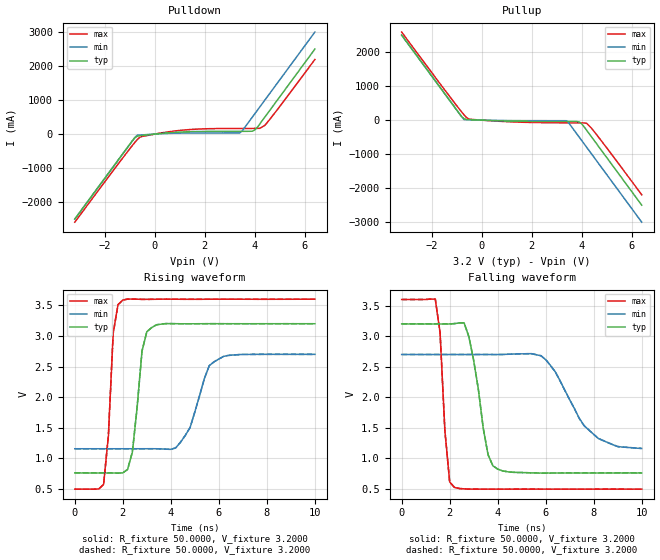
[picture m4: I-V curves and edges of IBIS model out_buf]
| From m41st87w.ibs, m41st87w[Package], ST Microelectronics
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|   Model out_buf
[Model]   out_buf
Model_type   Output
Polarity   Non-Inverting
Vmeas =   1.5000V
Cref =  50.0000pF
Rref =   0.6450k
Vref =   1.7500V
C_comp   9.2400pF   8.7300pF   9.7600pF
[Temperature Range]   27.0000   85.0000   -40.0000
[Voltage Range]   3.2000V   2.7000V   3.6000V
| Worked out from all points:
|   slope of the pulldown table from 0 to 0.48 V, typ, clamps not added: 14.3 ohm
|   slope of the pullup table from 0 to 0.48 V, typ, clamps not added: 36.1 ohm
|   rising waveform, R_fixture 50.0000, V_fixture 3.2000: 20-80 % time 352ps typ, 738ps min, 255ps max; typ from 0.763 V to 3.2 V
|   rising waveform, R_fixture 50.0000, V_fixture 3.2000: 20-80 % time 352ps typ, 738ps min, 255ps max; typ from 0.763 V to 3.2 V
|   falling waveform, R_fixture 50.0000, V_fixture 3.2000: 20-80 % time 568ps typ, 1.35ns min, 271ps max; typ from 3.2 V to 0.763 V
|   falling waveform, R_fixture 50.0000, V_fixture 3.2000: 20-80 % time 568ps typ, 1.35ns min, 271ps max; typ from 3.2 V to 0.763 V
[Pulldown]
| voltage   I(typ)   I(min)   I(max)
-3.2V     -2.5A      -2.5A      -2.591A
-900mV    -200mA     -200mA     -337.2mA
-700mV    -62.82mA   -32.69mA   -160.6mA
-500mV    -39.9mA    -23.29mA   -67.68mA
900mV     54.82mA    27.57mA    99.9mA
3.4V      81.17mA    34.99mA    165.9mA
3.5V      81.34mA    100mA      166.2mA
3.9V      85.33mA    500mA      167.5mA
4V        121.5mA    600mA      167.8mA
4.2V      300mA      800mA      168.7mA
4.4V      500mA      1A         256.9mA
6.4V      2.5A       3A         2.194A
[Pullup]
| voltage   I(typ)   I(min)   I(max)
-3.2V     2.5A       2.5A       2.589A
-900mV    200mA      200mA      332.4mA
-700mV    40.85mA    13.49mA    150.9mA
-500mV    16.27mA    9.076mA    29.84mA
-300mV    9.6mA      5.337mA    16.43mA
1.4V      -30.11mA   -14.05mA   -55.76mA
3.4V      -38.98mA   -17.38mA   -78.6mA
3.9V      -52.76mA   -500mA     -80.59mA
4V        -109mA     -600mA     -80.96mA
4.2V      -300mA     -800mA     -95.49mA
4.6V      -700mA     -1.2A      -430.6mA
6.4V      -2.5A      -3A        -2.194A
[Ramp]
| variable   typ   min   max
dV/dt_r   1.8251/0.5037n   1.4741/1.0410n   2.0984/0.2774n
dV/dt_f   1.8833/0.3740n   1.5639/0.8009n   2.1365/0.1990n
R_load = 0.6450k
[Rising Waveform]
R_fixture = 50.0000
V_fixture = 3.2000
V_fixture_min = 2.7000
V_fixture_max = 3.6000
| time   V(typ)   V(min)   V(max)
0s        762.9mV    1.158V     498.2mV
1.2ns     762.9mV    1.158V     576.1mV
1.6ns     762.9mV    1.158V     3.047V
2ns       763.6mV    1.158V     3.587V
2.4ns     1.105V     1.158V     3.603V
2.8ns     2.755V     1.158V     3.598V
3.2ns     3.136V     1.159V     3.599V
4.4ns     3.199V     1.263V     3.6V
5.8ns     3.201V     2.579V     3.6V
10ns      3.2V       2.7V       3.6V
[Rising Waveform]
R_fixture = 50.0000
V_fixture = 3.2000
V_fixture_min = 2.7000
V_fixture_max = 3.6000
| time   V(typ)   V(min)   V(max)
0s        762.9mV    1.158V     498.2mV
1.2ns     762.9mV    1.158V     576.1mV
1.6ns     762.9mV    1.158V     3.047V
2ns       763.6mV    1.158V     3.587V
2.4ns     1.105V     1.158V     3.603V
2.8ns     2.755V     1.158V     3.598V
3.2ns     3.136V     1.159V     3.599V
4.4ns     3.199V     1.263V     3.6V
5.8ns     3.201V     2.579V     3.6V
10ns      3.2V       2.7V       3.6V
[Falling Waveform]
R_fixture = 50.0000
V_fixture = 3.2000
V_fixture_min = 2.7000
V_fixture_max = 3.6000
| time   V(typ)   V(min)   V(max)
0s        3.2V       2.7V       3.6V
1.4ns     3.2V       2.7V       3.606V
1.6ns     3.2V       2.7V       3.058V
2ns       3.2V       2.7V       615.7mV
2.2ns     3.206V     2.7V       526.7mV
2.8ns     2.991V     2.7V       499.3mV
3.8ns     880.8mV    2.7V       498.1mV
5.8ns     762mV      2.681V     498.2mV
7.6ns     763.1mV    1.536V     498.2mV
10ns      763mV      1.164V     498.1mV
[Falling Waveform]
R_fixture = 50.0000
V_fixture = 3.2000
V_fixture_min = 2.7000
V_fixture_max = 3.6000
| time   V(typ)   V(min)   V(max)
0s        3.2V       2.7V       3.6V
1.4ns     3.2V       2.7V       3.606V
1.6ns     3.2V       2.7V       3.058V
2ns       3.2V       2.7V       615.7mV
2.2ns     3.206V     2.7V       526.7mV
2.8ns     2.991V     2.7V       499.3mV
3.8ns     880.8mV    2.7V       498.1mV
5.8ns     762mV      2.681V     498.2mV
7.6ns     763.1mV    1.536V     498.2mV
10ns      763mV      1.164V     498.1mV
